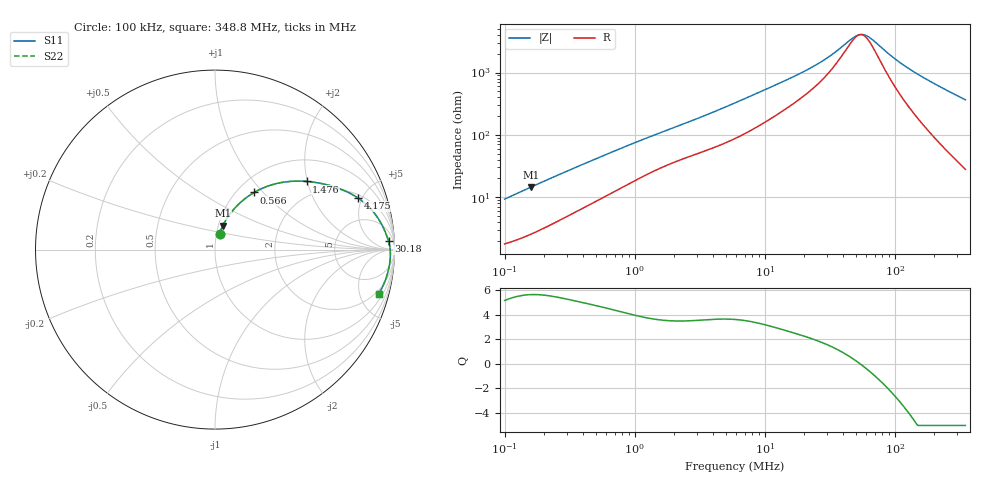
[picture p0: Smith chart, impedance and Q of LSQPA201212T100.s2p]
! LSQPA201212T100  S-PARAMETER MODEL  ( General Type )
! Model Generated by TAIYO YUDEN Corporation (http://www.ty-top.com)
! Version 2.0
! TAIYO YUDEN Control No. 100810NF25SB-FKC
! Copyright(c) 2007 TAIYO YUDEN CO.,LTD. All Rights Reserved.
! Product Description (link to TY-COMPAS)
! https://ds.yuden.co.jp/TYCOMPAS/or/detail?pn=LSQPA201212T100K&u=M
! Products Name : Inductors
! Characteristics :
!  Inductance : 10 uH , SRF(min) : 40 MHz , DC Resistance(max) : 1.56 Ohm
!  Rated Current : Saturation :240 mA , Temp Rise : 340 mA (40 degC)
!  Case Size : 2.0 x 1.25 / 0.079 x 0.049 [mm/inch] , Thickness : 1.25 / 0.049 [mm/inch]
!  (Conditions: Temperature = 25 degC , DC Bias Current/Voltage = 0A / 0V)
! External Node Assignments :
!  1  o---GGG---o  2
! GND o---------o GND
! Frequency Range : 0.1MHz  -  348.750116MHz  [ 402 STEP ]
# MHz S RI R 50
! Freq[MHz].  S11 Real  S11 Imag  S21 Real  S21 Imag  S12 Real  S12 Imag  S22 Real  S22 Imag
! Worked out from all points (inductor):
!   401 points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, 100 kHz to 348.8 MHz, reference 50 ohm
!   read as one part in series: L = 14.4 uH near 104.2 kHz
!   highest Q = 5.62 at 159.8 kHz (marker M1), where L = 14.3 uH
!   self-resonance near 54.08 MHz
!   S11 on the Smith chart (normalised r, x): 100 kHz: 1.04, +0.18; 566 kHz: 1.19, +0.89; 1.476 MHz: 1.55, +1.98; 4.175 MHz: 2.28, +4.61; 30.18 MHz: 20, +29; 348.8 MHz: 1.56, -7.27
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0.1  0.0253 0.0875  0.9747 -0.0875  0.9747 -0.0875  0.0253 0.0875
0.159843  0.0435 0.1336  0.9565 -0.1336  0.9565 -0.1336  0.0435 0.1336
0.255499  0.0808 0.1953  0.9192 -0.1953  0.9192 -0.1953  0.0808 0.1953
0.392077  0.1407 0.2616  0.8593 -0.2616  0.8593 -0.2616  0.1407 0.2616
0.565958  0.2184 0.3185  0.7816 -0.3185  0.7816 -0.3185  0.2184 0.3185
0.923284  0.3595 0.3716  0.6405 -0.3716  0.6405 -0.3716  0.3595 0.3716
1.475808  0.5101 0.3799  0.4899 -0.3799  0.4899 -0.3799  0.5101 0.3799
1.537242  0.5229 0.3788  0.4771 -0.3788  0.4771 -0.3788  0.5229 0.3788
2.507802  0.6677 0.3488  0.3323 -0.3488  0.3323 -0.3488  0.6677 0.3488
4.175421  0.7953 0.2882  0.2047 -0.2882  0.2047 -0.2882  0.7953 0.2882
5.905507  0.8596 0.2352  0.1404 -0.2352  0.1404 -0.2352  0.8596 0.2352
13.35084  0.938 0.1218  0.062 -0.1218  0.062 -0.1218  0.938 0.1218
23.15412  0.9602 0.068  0.0398 -0.068  0.0398 -0.068  0.9602 0.068
30.18284  0.9672 0.046  0.0328 -0.046  0.0328 -0.046  0.9672 0.046
47.27139  0.9747 0.0107  0.0253 -0.0107  0.0253 -0.0107  0.9747 0.0107
54.52458  0.976 -0.000651  0.024 0.000651  0.024 0.000651  0.976 -0.000651
59.15854  0.9765 -0.00723  0.0235 0.00723  0.0235 0.00723  0.9765 -0.00723
64.18634  0.9769 -0.0139  0.0231 0.0139  0.0231 0.0139  0.9769 -0.0139
90.78195  0.9766 -0.0444  0.0234 0.0444  0.0234 0.0444  0.9766 -0.0444
118.3399  0.9741 -0.0712  0.0259 0.0712  0.0259 0.0712  0.9741 -0.0712
160.6851  0.9676 -0.1081  0.0324 0.1081  0.0324 0.1081  0.9676 -0.1081
348.7501  0.9139 -0.2447  0.0861 0.2447  0.0861 0.2447  0.9139 -0.2447
